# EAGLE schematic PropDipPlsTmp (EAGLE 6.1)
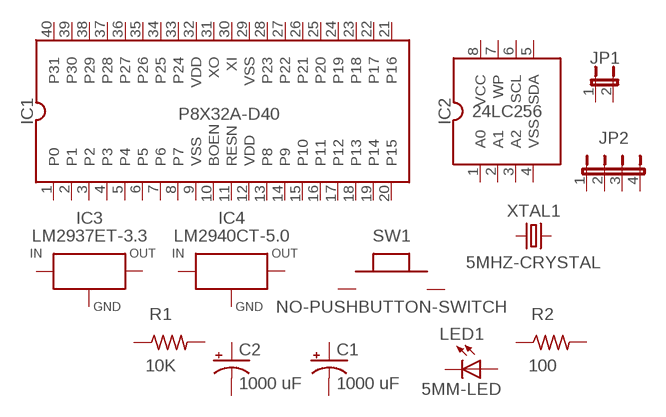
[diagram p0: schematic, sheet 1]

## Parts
C1  UVR0J102MPD  [UVR0J102MPD]
C2  UVR0J102MPD  [UVR0J102MPD]
IC1  P8X32A-D40DIP-40  [P8X32A-D40]
IC2  24LC256DIP-8  [24LC256]
IC3  LM2937ET-3.3TO-220  [LM2937ET-3.3]
IC4  LM2940CT-5.0  [LM2940CT-5.0]
JP1  2-PIN-HEADER  [2-PIN-HEADER]
JP2  4-PIN-HEADER  [4-PIN-HEADER]
LED1  5MM-LED  [5MM-LED]
R1  10K-OHM-RESISTOR  [10K-OHM-RESISTOR]
R2  100-OHM-RESISTOR  [100-OHM-RESISTOR]
SW1  NO-PUSHBUTTON-SWITCH  [NO-PUSHBUTTON-SWITCH]
XTAL1  5MHZ-CRYSTAL  [5MHZ-CRYSTAL]
Unconnected: C1.P$1(+) C1.P$2(-) C2.P$1(+) C2.P$2(-) IC1.1(P0) IC1.2(P1) IC1.3(P2) IC1.4(P3) IC1.5(P4) IC1.6(P5) IC1.7(P6) IC1.8(P7) IC1.10(BOEN) IC1.11(RESN) IC1.13(P8) IC1.14(P9) IC1.15(P10) IC1.16(P11) IC1.17(P12) IC1.18(P13) IC1.19(P14) IC1.20(P15) IC1.21(P16) IC1.22(P17) IC1.23(P18) IC1.24(P19) IC1.25(P20) IC1.26(P21) IC1.27(P22) IC1.28(P23) IC1.30(XI) IC1.31(XO) IC1.33(P24) IC1.34(P25) IC1.35(P26) IC1.36(P27) IC1.37(P28) IC1.38(P29) IC1.39(P30) IC1.40(P31) IC2.1(A0) IC2.2(A1) IC2.3(A2) IC2.5(SDA) IC2.6(SCL) IC2.7(WP) JP1.1 JP1.2 JP2.1 JP2.2 JP2.3 JP2.4 LED1.A LED1.K(C) R1.1 R1.2 R2.1 R2.2 SW1.P$1 SW1.P$2 SW1.P$3 SW1.P$4 XTAL1.1 XTAL1.2

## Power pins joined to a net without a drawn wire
GND: IC3.GND IC4.GND
IN: IC3.IN IC4.IN
OUT: IC3.OUT IC4.OUT
VCC: IC2.8(VCC)
VDD: IC1.12(VDD) IC1.32(VDD)
VSS: IC1.9(VSS) IC1.29(VSS) IC2.4(VSS)

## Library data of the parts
C1 C2 = propeller-dip-plus:UVR0J102MPD: 6.3V 1000 µF Electrolytic Capacitor
IC1 = propeller-dip-plus:P8X32A-D40: Parallax Propeller P8X32A-D40 Microcontroller DIP40
IC2 = propeller-dip-plus:24LC256: 256 Kbit (32 KByte) Industrial I2C Serial EEPROM
IC3 = propeller-dip-plus:LM2937ET-3.3: 3.3V 500mA Voltage Regulator
IC4 = propeller-dip-plus:LM2940CT-5.0: 5V 1A Low Droput Regulator
JP1 = propeller-dip-plus:2-PIN-HEADER: 2 Pin Header
JP2 = propeller-dip-plus:4-PIN-HEADER: 4 Pin Header
LED1 = propeller-dip-plus:5MM-LED: Green 5MM LED (T-1 3/4)
R1 = propeller-dip-plus:10K-OHM-RESISTOR: 1/4 Watt 10K Ohm Resistor
R2 = propeller-dip-plus:100-OHM-RESISTOR: 1/4 Watt 100 Ohm Resistor
SW1 = propeller-dip-plus:NO-PUSHBUTTON-SWITCH: Normally Open Pushbutton Tact Switch
XTAL1 = propeller-dip-plus:5MHZ-CRYSTAL: HC-49US 5MHz Quartz Crystal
